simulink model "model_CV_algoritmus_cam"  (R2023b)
settings: Solver=FixedStepAuto  StartTime=0.0  StopTime=inf  RelTol=1e-3  EnableMultiTasking=on
undefined symbols (not defined in the file): adaptor, C, Camera, genericvideo, HD, HP, imaq, MATLAB, Newmine, none, ProgramData, R2023b, SupportPackages, supportpackages, toolbox, videoinput, win64, winvideo
libraries: visionsinks x2, imaqlib x1, deeplib x1, visiontextngfix x1, dspstat3 x1

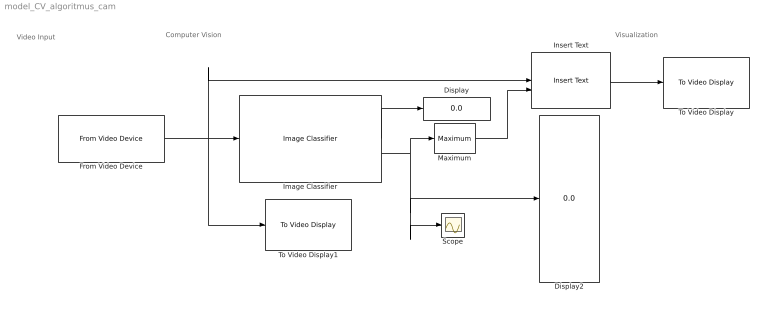
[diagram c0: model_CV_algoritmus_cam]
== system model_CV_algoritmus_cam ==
  note: Video Input
  note: Computer Vision
  note: Visualization
  Display : Display
  Display2 : Display
  From Video Device : imaqlib/From Video Device  DeviceMenu=winvideo 1 (HP HD Camera)  Device=winvideo 2 (Newmine Camera)  ObjConstructor=videoinput('winvideo', 2)  VideoFormatMenu=MJPG_320x240  VideoFormat=MJPG_320x240  VideoSource=input1  ROIPosition=[0 0 240 320]  EnableHWTrigger=off  TriggerConfiguration=none/none  SampleTime=1/10  OutputPortsMode=One multidimensional signal  DataType=uint8  CanDoHWTrigger=no  ReturnedColorSpace=rgb  BlockHandle=214.0046  ROIWidth=320  ROIHeight=240  ROIColumn=0  ROIRow=0  EngXMLPath=C:\Program Files\MATLAB\R2023b\toolbox\imaq\imaq\private  DevXMLPath=C:\ProgramData\MATLAB\SupportPackages\R2023b\toolbox\imaq\supportpackages\genericvideo\adaptor\win64  EngLibPath=C:\Program Files\MATLAB\R2023b\toolbox\imaq\imaqblks\imaqmex\win64  ColorSpace=rgb  BayerSensorAlignment=grbg  ImaqMode=off
  Image Classifier : deeplib/Image Classifier  Network=Network from MAT-file  NetworkFunction=squeezenet  NetworkFilePath=trainedNetwork.mat  MiniBatchSize=8  ResizeInput=on  Classification=on  Predictions=on  ForceInterpretedSim=off  PredictMode=All probabilities and labels  K=5
  Insert Text : visiontextngfix/Insert Text  inputType=Obsolete  theText={'Hmozdinka','Hrebik','Matice','Matice kridlova','Podlozka','Prazdne','Sroub','Vrut'}  getTextLocFrom=Specify via dialog  textLoc=[1 1]  getTextColorFrom=Specify via dialog  textColor=[0 0 0]  getTextIntensityFrom=Specify via dialog  textIntensity=0  getTextOpacityFrom=Specify via dialog  textOpacity=1.0  dummyVar2=0  dummyVar3=0  dummyVar4=0  imagePorts=One multidimensional signal  isInputTransposed=off  fontFace=LucidaSansRegular  dummyVar1=0  blockFontSize=32  antiAliased=on
  Maximum : dspstat3/Maximum  operation=maximum  fcn=Index  indexBase=One  operateOver=Each row  Dimension=1  InputProcessing=Columns as channels (frame based)  reset=None  roiEnable=off  roiType=Rectangles  roiPortion=Entire ROI  roiOutput=Individual statistics for each ROI  roiFlag=off  roundingMode=Floor  overflowMode=off  accumDataTypeStr=Inherit: Same as product output  accumLastDataTypeStr=Inherit: Same as product output
  Scope : Scope
  To Video Display : visionsinks/To Video Display  windowSizeMode=Normal  openAtMdlStart=on  fullScreen=off  videoWindowX=1368  videoWindowY=406  saveWindowSize=off  videoWindowWidth=227  videoWindowHeight=227  inputColorFormat=RGB  inputType=Obsolete  imagePorts=One multidimensional signal  OutputDevice=On-screen video monitor  dataOrg=Column-major  isWindowOpen=off
  To Video Display1 : visionsinks/To Video Display  windowSizeMode=Normal  openAtMdlStart=on  fullScreen=off  videoWindowX=1135  videoWindowY=406  saveWindowSize=off  videoWindowWidth=227  videoWindowHeight=227  inputColorFormat=RGB  inputType=Obsolete  imagePorts=One multidimensional signal  OutputDevice=On-screen video monitor  dataOrg=Column-major  isWindowOpen=off
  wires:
  From Video Device/1 -> Image Classifier/1, Insert Text/1, To Video Display1/1
  Image Classifier/1 -> Display/1
  Image Classifier/2 -> Maximum/1, Scope/1, Display2/1
  Insert Text/1 -> To Video Display/1
  Maximum/1 -> Insert Text/2
